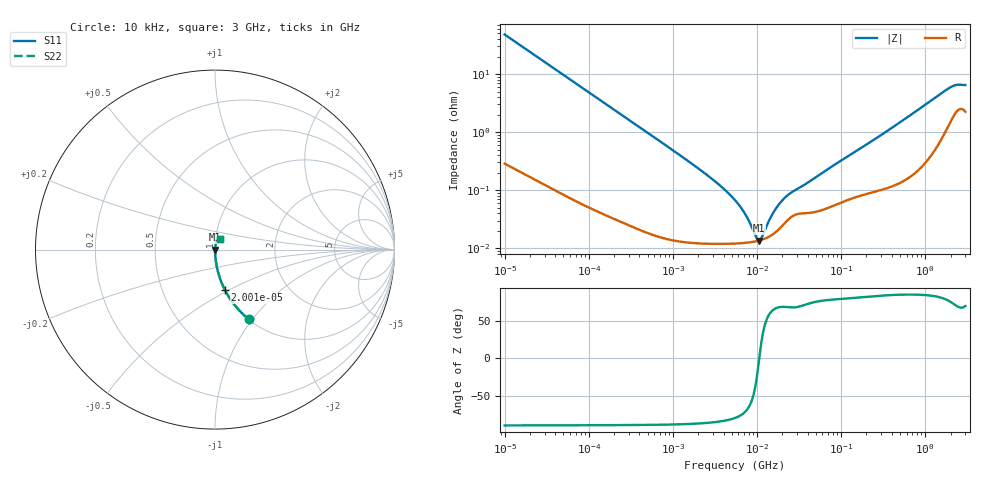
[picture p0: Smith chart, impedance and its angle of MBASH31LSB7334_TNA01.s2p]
! MBASH31LSB7334_TNA01  S-PARAMETER MODEL  ( Standard Model )
! Model Generated by TAIYO YUDEN Corporation (http://www.ty-top.com)
! Version 1.0
! TAIYO YUDEN Control No. 220601
! Copyright(c) 2013 TAIYO YUDEN CO.,LTD. All Rights Reserved.
! Product Description (link to TY-COMPAS)
! https://ds.yuden.co.jp/TYCOMPAS/or/detail?pn=MBASH31LSB7334KTNA01&u=M
! Products Name : Multilayer Ceramic Capacitors
! Characteristics :
!  Capacitance : 0.33 [uF] , Rated Voltage : 100 [V] , TCC : X7R
!  Case Size : 3.2 x 1.6 / 0.126 x 0.063 [mm/inch] , Thickness : 1.6 / 0.063 [mm/inch]
!  (Conditions: Temperature = 25 [degC] , DC Bias Voltage = 0 [V])
! External Node Assignments :
!  1  o---| |---o  2
! GND o---------o GND
! Frequency Range : 10kHz  -  3GHz  [ 401 STEP ]
# MHZ S RI R 50
! Freq[MHz].  S11 Real  S11 Imag  S21 Real  S21 Imag  S12 Real  S12 Imag  S22 Real  S22 Imag
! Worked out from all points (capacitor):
!   401 points, 10 kHz to 3 GHz, reference 50 ohm
!   read as one part in series: C = 331 nF near 10.65 kHz
!   lowest |Z| = 13.6 mohm at 10.62 MHz (marker M1)
!   series resonance near 10.65 MHz, so ESL is about 670 pH
!   S11 on the Smith chart (normalised r, x): 10 kHz: 1.01, -0.96; 20.01 kHz: 1.00, -0.48; 3 GHz: 1.04, +0.12
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0.01  0.1885 -0.3882  0.8115 0.3882  0.8115 0.3882  0.1885 -0.3882
0.02001  0.056 -0.2265  0.944 0.2265  0.944 0.2265  0.056 -0.2265
0.038796  0.0162 -0.1222  0.9838 0.1222  0.9838 0.1222  0.0162 -0.1222
0.082683  0.00399 -0.0583  0.996 0.0583  0.996 0.0583  0.00399 -0.0583
0.683653  0.000208 -0.00714  0.9998 0.00714  0.9998 0.00714  0.000208 -0.00714
2.737278  0.000122 -0.00168  0.9999 0.00168  0.9999 0.00168  0.000122 -0.00168
4.124064  0.00012 -0.00102  0.9999 0.00102  0.9999 0.00102  0.00012 -0.00102
5.477226  0.000121 -0.000663  0.9999 0.000663  0.9999 0.000663  0.000121 -0.000663
7.048603  0.000123 -0.000394  0.9999 0.000394  0.9999 0.000394  0.000123 -0.000394
7.996027  0.000126 -0.00027  0.9999 0.00027  0.9999 0.00027  0.000126 -0.00027
9.6612  0.000132 -9.1e-05  0.9999 9.1e-05  0.9999 9.1e-05  0.000132 -9.1e-05
10.61963  0.000136 -2.44e-06  0.9999 2.44e-06  0.9999 2.44e-06  0.000136 -2.44e-06
11.67315  0.000142 8.65e-05  0.9999 -8.65e-05  0.9999 -8.65e-05  0.000142 8.65e-05
13.66633  0.000156 0.000238  0.9998 -0.000238  0.9998 -0.000238  0.000156 0.000238
15.50326  0.000175 0.000363  0.9998 -0.000363  0.9998 -0.000363  0.000175 0.000363
19.95104  0.000243 0.00062  0.9998 -0.00062  0.9998 -0.00062  0.000243 0.00062
24.87798  0.000335 0.000821  0.9997 -0.000821  0.9997 -0.000821  0.000335 0.000821
45.28751  0.000414 0.00146  0.9996 -0.00146  0.9996 -0.00146  0.000414 0.00146
374.4521  0.00124 0.011  0.9988 -0.011  0.9988 -0.011  0.00124 0.011
1929.399  0.0165 0.0542  0.9835 -0.0542  0.9835 -0.0542  0.0165 0.0542
2331.196  0.025 0.0582  0.975 -0.0582  0.975 -0.0582  0.025 0.0582
3000  0.0253 0.0577  0.9747 -0.0577  0.9747 -0.0577  0.0253 0.0577
